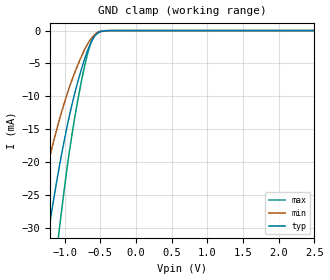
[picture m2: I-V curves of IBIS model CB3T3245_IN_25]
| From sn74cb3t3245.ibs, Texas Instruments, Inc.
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[Model]   CB3T3245_IN_25
Model_type  Input
Vinl=0.7
Vinh=1.7
| variable   typ   min   max
C_comp   2.67pF   1.96pF   3.04pF
[Temperature Range]   40   100   -40
| Ambient temperature   25   85   -40
[Voltage range]   2.5   2.3   2.7
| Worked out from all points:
|   GND clamp passes 1 mA (typ) near -0.59 V on its own axis
[GND Clamp]
| CB3T3245_IN_25
|   Voltage   I(typ)   I(min)   I(max)
-5V       -417.4mA   -313.8mA   -530.2mA
-1.47V    -49.2mA    -32.32mA   -71.86mA
-1.425V   -45.58mA   -29.9mA    -66.75mA
-1.23V    -30.96mA   -20.24mA   -45.61mA
-1.075V   -20.82mA   -13.68mA   -30.43mA
-935mV    -13.11mA   -8.72mA    -18.64mA
-790mV    -6.857mA   -4.6mA     -9.175mA
-665mV    -2.695mA   -1.819mA   -3.051mA
-605mV    -1.322mA   -915.9uA   -1.222mA
-545mV    -493.3uA   -373.5uA   -325.8uA
-345mV    -3.226uA   -4.882uA   -349.1nA
2.5V      96.07pA    415.1pA    20.34pA
